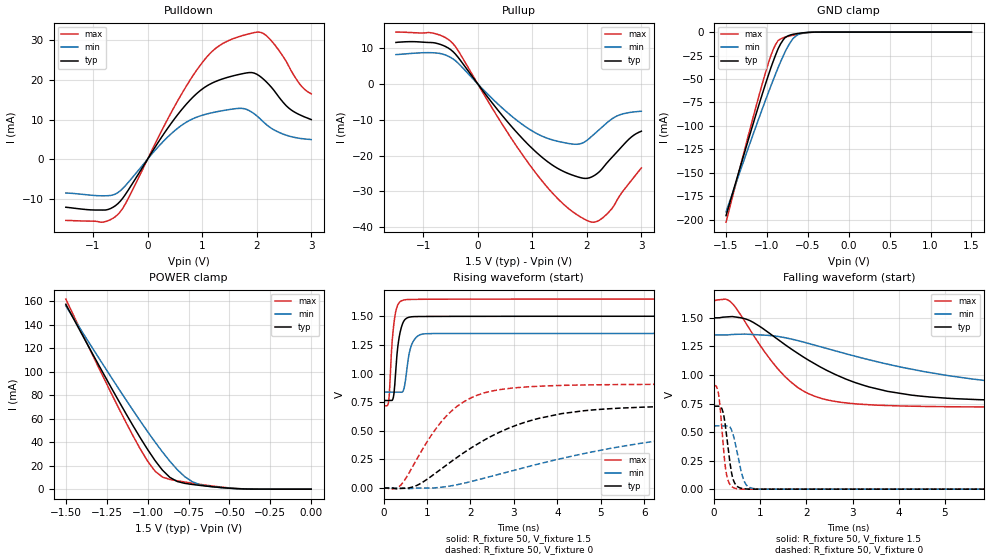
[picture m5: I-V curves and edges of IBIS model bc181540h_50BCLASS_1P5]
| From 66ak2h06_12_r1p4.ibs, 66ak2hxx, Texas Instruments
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|   Model Cell bc181540h_50BCLASS_1P5
|bc181540h_50BCLASS_1P5
[Model]   bc181540h_50BCLASS_1P5
Model_type   I/O
Polarity   Non-Inverting
Enable   Active-Low
Vinl =  0.525
Vinh =  0.975
Cref =  15.0000pF
Rref =  100.0000M
Vref =  0V
Vmeas =  0.75
C_comp   1.17072p   0.570099p   1.17447p
[Model Spec]
Vinl   0.525   0.4725   0.5775
Vinh   0.975   0.8775   1.0725
[Temperature Range]   25   125   -40
[Voltage Range]   1.5   1.35   1.65
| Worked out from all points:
|   slope of the pulldown table from 0 to 0.225 V, typ, clamps not added: 46 ohm
|   slope of the pullup table from 0 to 0.225 V, typ, clamps not added: 49.6 ohm
|   GND clamp passes 1 mA (typ) near -0.58 V on its own axis
|   POWER clamp passes 1 mA (typ) near -0.52 V on its own axis
|   rising waveform, R_fixture 50, V_fixture 1.5: 20-80 % time 117ps typ, 138ps min, 102ps max; typ from 0.764 V to 1.5 V
|   rising waveform, R_fixture 50, V_fixture 0: 20-80 % time 2.07ns typ, 4.43ns min, 1.08ns max; typ from 0 V to 0.727 V
|   falling waveform, R_fixture 50, V_fixture 1.5: 20-80 % time 1.98ns typ, 3.81ns min, 1.09ns max; typ from 1.5 V to 0.764 V
|   falling waveform, R_fixture 50, V_fixture 0: 20-80 % time 141ps typ, 181ps min, 119ps max; typ from 0.727 V to 0 V
[POWER_clamp]
|   voltage   I(typ)   I(min)   I(max)
-1.5V     157.2mA    155.9mA    161.7mA
-1.273V   98.95mA    106mA      95.87mA
-1.091V   54.38mA    67.4mA     45.82mA
-1V       33.74mA    48.95mA    23.8mA
-954.5mV  24.35mA    40.1mA     15.29mA
-909.1mV  16.14mA    31.61mA    10.28mA
-863.6mV  9.975mA    23.68mA    8.252mA
-818.2mV  6.508mA    16.53mA    7.086mA
-727.3mV  4mA        6.353mA    5.092mA
-681.8mV  3.231mA    3.88mA     4.159mA
-409.1mV  177.3uA    258.7uA    224.6uA
0V        677pA      15.94nA    186.8pA
[Pulldown]
|   voltage   I(typ)   I(min)   I(max)
-1.5V     -12.14mA   -8.55mA    -15.46mA
-818.2mV  -12.85mA   -9.261mA   -15.91mA
-500mV    -10.61mA   -7.974mA   -13.27mA
272.7mV   5.882mA    4.26mA     7.58mA
681.8mV   13.43mA    9.079mA    17.79mA
1.091V    18.52mA    11.41mA    25.87mA
1.409V    20.41mA    12.32mA    29.41mA
1.818V    21.77mA    12.54mA    31.48mA
2.136V    20.04mA    9.227mA    31.59mA
2.591V    12.86mA    5.83mA     23.38mA
2.818V    11.01mA    5.19mA     18.46mA
3V        9.99mA     4.94mA     16.47mA
[Pullup]
|   voltage   I(typ)   I(min)   I(max)
-1.5V     11.57mA    8.17mA     14.46mA
-818.2mV  11.51mA    8.683mA    14.16mA
-454.5mV  9.026mA    6.992mA    11.26mA
409.1mV   -8.072mA   -6.173mA   -10.31mA
909.1mV   -16.68mA   -12.29mA   -21.7mA
1.455V    -23.5mA    -15.98mA   -31.85mA
1.909V    -26.28mA   -16.59mA   -37.38mA
2.136V    -25.6mA    -14.02mA   -38.62mA
2.318V    -23mA      -11.54mA   -37.06mA
2.591V    -18.37mA   -8.72mA    -31.5mA
2.818V    -14.82mA   -7.92mA    -26.94mA
3V        -13.21mA   -7.64mA    -23.48mA
[GND_clamp]
|   voltage   I(typ)   I(min)   I(max)
-1.5V     -195.7mA   -191.7mA   -202.6mA
-1.227V   -114.7mA   -123.3mA   -110.1mA
-1.045V   -62.85mA   -79.19mA   -51.48mA
-954.5mV  -38.7mA    -58mA      -25.52mA
-893.9mV  -24.32mA   -44.5mA    -13.19mA
-863.6mV  -17.74mA   -37.93mA   -9.007mA
-772.7mV  -5.381mA   -20.03mA   -5.301mA
-681.8mV  -2.343mA   -6.948mA   -3.394mA
-621.2mV  -1.47mA    -2.783mA   -2.285mA
-560.6mV  -800.4uA   -1.037mA   -1.331mA
-348.5mV  -9.367uA   -19.45uA   -12.08uA
1.5V      677pA      908.2nA    87.75pA
[Ramp]
| variable   typ   min   max
dV/dt_f   0.448428/1.9911618n   0.312312/3.8250903n   0.56817/1.1011954n
dV/dt_r 0.44094588/2.0762983n   0.33627/4.4513251n  0.5501052/1.0812199n
R_load = 50
[Rising Waveform]
R_fixture = 50
V_fixture = 1.5
V_fixture_min = 1.35
V_fixture_max = 1.65
|   time   V(typ)   V(min)   V(max)
0s        764.1mV    837.8mV    717.7mV
117.2ps   764.2mV    837.7mV    761.7mV
182.8ps   763.6mV    837.7mV    1.207V
222ps     789mV      837.7mV    1.389V
275.8ps   1.008V     837.8mV    1.537V
341.1ps   1.278V     837.7mV    1.61V
480ps     1.467V     888.7mV    1.643V
638.2ps   1.495V     1.245V     1.647V
972.9ps   1.498V     1.347V     1.648V
16.71ns   1.5V       1.35V      1.65V
[Rising Waveform]
R_fixture = 50
V_fixture = 0
V_fixture_min = 0
V_fixture_max = 0
|   time   V(typ)   V(min)   V(max)
0s        0V         0V         0V
420.9ps   -3.331mV   0V         36.7mV
1.151ns   117.4mV    0V         490.3mV
1.601ns   243.4mV    21.93mV    685.6mV
2.066ns   362.4mV    61.59mV    796.8mV
2.665ns   486.7mV    121.5mV    858.8mV
3.549ns   606.3mV    208.4mV    888.5mV
4.559ns   672.8mV    296.8mV    899.8mV
8.005ns   720.6mV    479.5mV    906.5mV
16.72ns   726.8mV    554.6mV    906.8mV
[Falling Waveform]
R_fixture = 50
V_fixture = 1.5
V_fixture_min = 1.35
V_fixture_max = 1.65
|   time   V(typ)   V(min)   V(max)
0s        1.5V       1.35V      1.651V
253.2ps   1.507V     1.35V      1.664V
406.6ps   1.511V     1.355V     1.623V
778.2ps   1.476V     1.355V     1.399V
1.219ns   1.361V     1.345V     1.137V
1.785ns   1.198V     1.304V     899.8mV
2.673ns   996mV      1.206V     764.9mV
4.263ns   824.1mV    1.052V     726.5mV
7.228ns   771.4mV    901.6mV    718.3mV
16.71ns   764.1mV    837.8mV    717.7mV
[Falling Waveform]
R_fixture = 50
V_fixture = 0
V_fixture_min = 0
V_fixture_max = 0
|   time   V(typ)   V(min)   V(max)
0s        726.8mV    554.6mV    906.7mV
104.6ps   726.8mV    554.6mV    829.8mV
201.9ps   671.4mV    554.6mV    395.5mV
248.6ps   563.3mV    554.4mV    200.4mV
290.4ps   428.5mV    555mV      102.9mV
409.4ps   98.41mV    490.2mV    16.58mV
576ps     9.941mV    184.5mV    0V
698.5ps   2.461mV    39.1mV     0V
971.5ps   0V         0V         0V
16.72ns   0V         0V         0V
